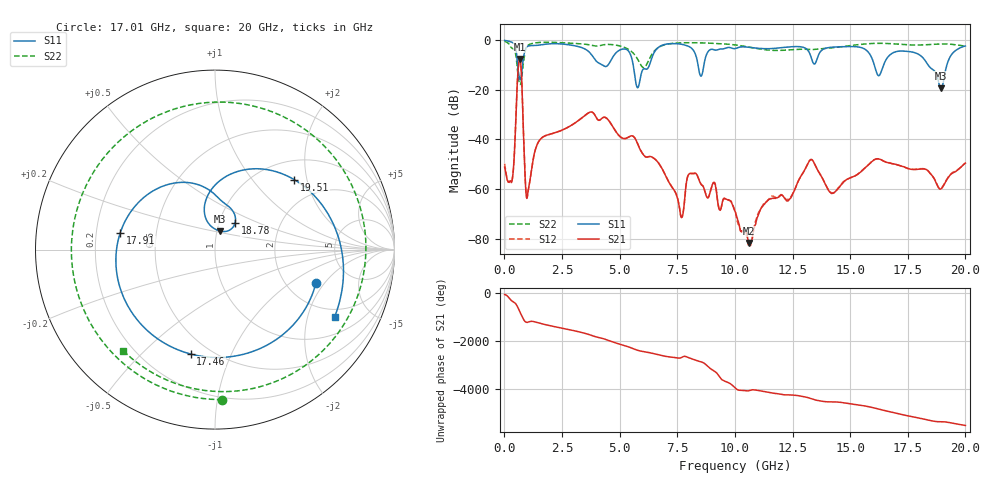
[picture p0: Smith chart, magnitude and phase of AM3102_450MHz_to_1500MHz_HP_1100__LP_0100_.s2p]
!Agilent Technologies,E8364B,MY43040894,A.07.50.67
!Agilent E8364B: A.07.50.67
!Date: Thursday, January 11, 2018 06:32:56
!Correction: S11(Full 2 Port(1,2))
!S21(Full 2 Port(1,2))
!S12(Full 2 Port(1,2))
!S22(Full 2 Port(1,2))
!S2P File: Measurements: S11, S21, S12, S22:
# Hz S  dB  R 50
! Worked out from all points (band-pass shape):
!   1601 points, 10 MHz to 20 GHz, reference 50 ohm
!   highest |S21| = -7.54 dB at 672.2 MHz (marker M1); lowest = -81.7 dB at 10.62 GHz (marker M2)
!   |S21| within 3 dB of the highest: 607.5 MHz to 720 MHz (112.4 MHz wide, 16.9 % of centre)
!   lowest |S11| = -19.4 dB at 18.94 GHz (marker M3), VSWR 1.24, Z = 51.9 + j10.8 ohm
!   |S11| at or under -10 dB: 5.589 GHz to 6.294 GHz (705.4 MHz wide, 11.9 % of centre); 16.05 GHz to 16.45 GHz (400.2 MHz wide, 2.46 % of centre); 18.38 GHz to 19.2 GHz (811 MHz wide, 4.32 % of centre)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
!   |S22| runs from -17.8 to -0.4 dB; largest |S21 - S12| = 0.0038
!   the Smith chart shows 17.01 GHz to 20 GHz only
!   S11 on the Smith chart (normalised r, x): 17.01 GHz: 2.88, -1.64; 17.46 GHz: 0.40, -0.72; 17.91 GHz: 0.30, +0.08; 18.78 GHz: 1.19, +0.37; 19.51 GHz: 1.41, +1.68; 20 GHz: 1.65, -2.98
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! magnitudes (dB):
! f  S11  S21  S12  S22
! 10 MHz  -0.1  -51.1  -49.8  -0.4
! 334.8 MHz  -0.9  -56.6  -56.3  -3.2
! 672.2 MHz  -15.7  -7.5  -7.5  -17.7
! 1.01 GHz  -2.4  -61.9  -62.3  -2.2
! 1.547 GHz  -1.9  -40.1  -40.0  -0.9
! 3.346 GHz  -2.9  -31.4  -31.4  -1.5
! 5.782 GHz  -19.1  -41.8  -41.8  -7.7
! 6.682 GHz  -2.9  -49.4  -49.4  -3.0
! 7.681 GHz  -1.6  -71.5  -71.3  -1.0
! 8.143 GHz  -3.4  -53.7  -53.7  -1.0
! 10.01 GHz  -3.4  -68.9  -68.7  -1.9
! 10.62 GHz  -2.8  -81.7  -82.5  -2.8
! 13.34 GHz  -7.8  -48.2  -48.1  -3.8
! 14.22 GHz  -2.8  -61.7  -61.6  -3.1
! 16.68 GHz  -6.4  -49.5  -49.3  -1.3
! 17.01 GHz  -4.5  -50.1  -50.1  -1.5
! 17.46 GHz  -4.5  -51.5  -51.5  -1.8
! 17.91 GHz  -5.4  -52.0  -51.9  -1.9
! 18.78 GHz  -14.6  -58.4  -58.2  -1.6
! 18.94 GHz  -19.4  -59.9  -59.7  -1.5
! 19.51 GHz  -4.6  -53.2  -52.9  -1.8
! 20 GHz  -2.3  -49.5  -49.5  -2.4
